{attribute 'Tc2GvlVarNames'}
VAR_GLOBAL
	sRecData				: ST_RecData;
	sMacData				: ST_MachineData;

(*临时变量, 和设置的参数比较, 参数修改后, 延时自动保存参数*)
(*结构体类型(数组长度)必须一致, 否则比较/复制时, 会有意想不到的错误*)
	_sRecData				: ST_RecData;
	_sMacData				: ST_MachineData;
END_VAR
